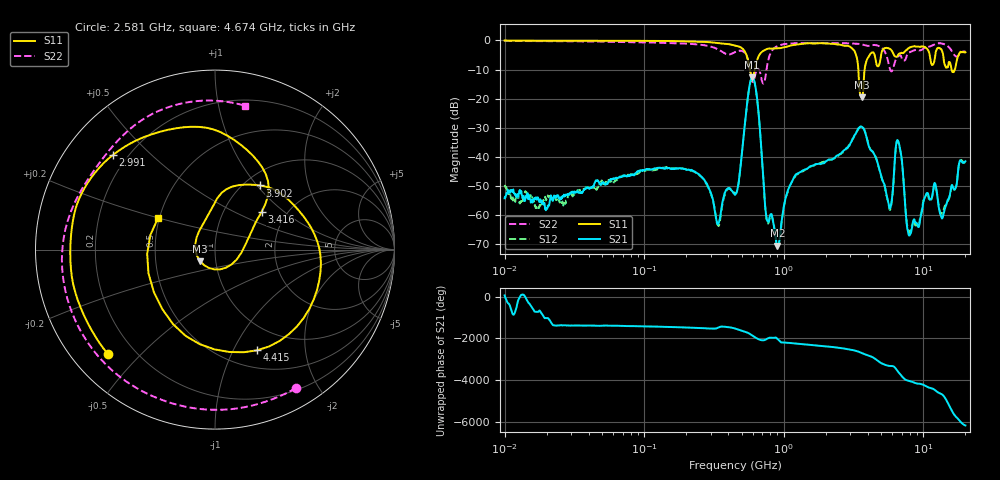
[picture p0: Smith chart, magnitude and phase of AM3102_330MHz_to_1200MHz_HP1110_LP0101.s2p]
! Date/Time: Tue, Sep 11, 2018 5:23 PM
! Network Analyzer: Agilent Technologies E8362B Rev: A.07.50.63
! Sweep from 0.010 to 20.000 GHz, 1601 Points, Sweep Type: LOG
! Power Supply: 4.949 V, 0.001 A
# Hz S DB R 50
!freq MagS11 AngS11 MagS21 AngS21 MagS12 AngS12 MagS22 AngS22
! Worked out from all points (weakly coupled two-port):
!   1601 points, 10 MHz to 20 GHz, reference 50 ohm
!   highest |S21| = -12.68 dB at 594.7 MHz (marker M1); lowest = -70.4 dB at 899.1 MHz (marker M2)
!   lowest |S11| = -19.6 dB at 3.617 GHz (marker M3), VSWR 1.23, Z = 42.1 - j5.58 ohm
!   |S11| at or under -10 dB: 572.1 MHz to 620.5 MHz (48.43 MHz wide, 8.12 % of centre); 3.421 GHz to 3.792 GHz (371 MHz wide, 10.3 % of centre); 15.92 GHz to 16.8 GHz (886.5 MHz wide, 5.42 % of centre)
!   |S22| runs from -14.8 to -0.2 dB; largest |S21 - S12| = 0.0052
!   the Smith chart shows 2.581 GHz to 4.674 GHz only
!   S11 on the Smith chart (normalised r, x): 2.581 GHz: 0.11, -0.40; 2.991 GHz: 0.15, +0.39; 3.416 GHz: 1.50, +0.71; 3.902 GHz: 1.18, +1.04; 4.415 GHz: 0.70, -1.24; 4.674 GHz: 0.49, +0.20
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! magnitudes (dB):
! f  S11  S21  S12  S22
! 10 MHz  0.0  -54.2  -49.6  -0.2
! 35.55 MHz  -0.1  -52.2  -51.4  -0.4
! 126.4 MHz  -0.2  -43.7  -44.1  -0.8
! 255.3 MHz  -0.5  -46.6  -46.7  -1.5
! 337.9 MHz  -1.0  -63.1  -63.5  -3.1
! 447.2 MHz  -1.8  -53.0  -52.5  -4.0
! 594.7 MHz  -12.4  -12.7  -12.8  -14.1
! 750.6 MHz  -3.0  -60.6  -61.1  -10.3
! 899.1 MHz  -2.7  -70.4  -70.5  -2.0
! 1.124 GHz  -1.8  -49.3  -49.2  -1.1
! 1.59 GHz  -1.0  -43.0  -43.0  -0.9
! 2.581 GHz  -1.6  -38.8  -38.8  -1.0
! 2.991 GHz  -2.2  -35.5  -35.4  -1.0
! 3.416 GHz  -9.5  -30.2  -30.5  -1.2
! 3.617 GHz  -19.6  -29.6  -29.4  -1.4
! 3.902 GHz  -7.2  -32.9  -32.9  -1.8
! 4.415 GHz  -4.3  -38.8  -38.7  -1.6
! 4.674 GHz  -8.8  -41.6  -41.7  -1.7
! 5.652 GHz  -2.7  -56.3  -56.6  -8.2
! 6.549 GHz  -5.3  -34.2  -34.5  -5.6
! 7.958 GHz  -2.5  -66.9  -65.8  -4.1
! 20 GHz  -4.1  -41.5  -42.0  -3.8
